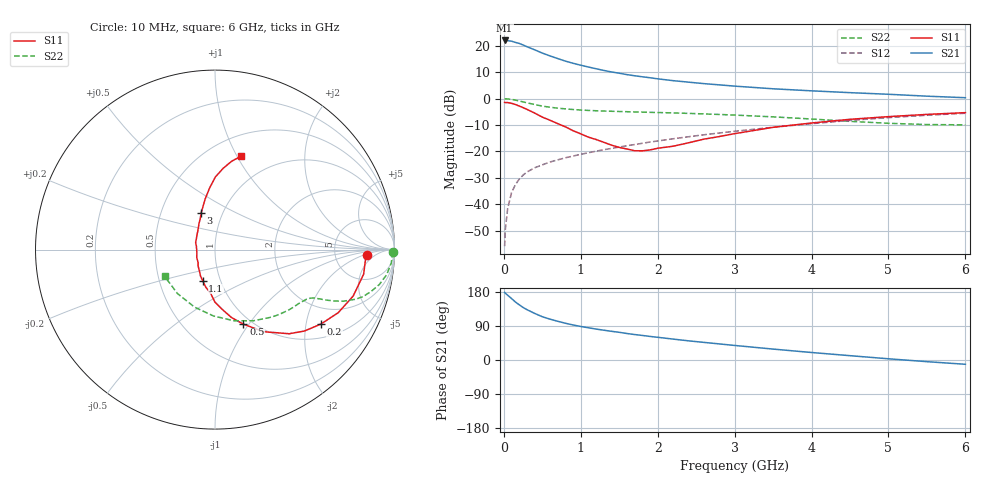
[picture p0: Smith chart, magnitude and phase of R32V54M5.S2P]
! SIEMENS Small Signal Semiconductors
! BFR181
! Si NPN RF Bipolar Junction Transistor in SOT23
! VCE = 2.5 V  IC = 4.5 mA
! Common Emitter S-Parameters:  May  1996
# GHz  S  MA  R  50
!  f  S11  S21  S12  S22
! GHz  MAG  ANG  MAG  ANG  MAG  ANG  MAG  ANG
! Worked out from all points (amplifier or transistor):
!   36 points, 10 MHz to 6 GHz, reference 50 ohm
!   highest |S21| = 22.0 dB at 10 MHz (marker M1)
!   |S21| within 3 dB of that: start of sweep to 354.1 MHz
!   unconditionally stable (mu >= 1): 1.156 GHz to 3.025 GHz
!   at 250 MHz: K = 0.39, MSG = 24.6 dB, |S12| = -29.0 dB
!   at 1.4 GHz: K = 1.05, MAG = 13.2 dB, |S12| = -18.9 dB
!   at 6 GHz: K = 0.86, MSG = 2.9 dB, |S12| = -5.6 dB
!   S11 on the Smith chart (normalised r, x): 10 MHz: 12, -2; 200 MHz: 1.41, -2.45; 500 MHz: 0.91, -0.94; 1.1 GHz: 0.82, -0.29; 3 GHz: 0.79, +0.34; 6 GHz: 0.71, +1.04
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0.01  0.8457 -1.9  12.61 178.2  0.0016 92.1  0.9919 -0.8
0.02  0.8404 -3.7  12.32 176.1  0.0034 87.3  0.9884 -1.7
0.05  0.8393 -9.4  12.48 170.9  0.0083 81.4  0.9852 -4.3
0.1  0.8121 -18.6  12.23 162.2  0.0165 81.3  0.9668 -8.3
0.15  0.7714 -27.1  11.57 153.1  0.0234 75.3  0.9359 -12.0
0.2  0.722 -35.0  11.09 145.7  0.0298 72.5  0.9005 -15.0
0.25  0.6739 -42.3  10.35 138.7  0.0355 69.3  0.8656 -17.6
0.3  0.625 -48.6  9.609 132.9  0.0406 67.5  0.8317 -19.4
0.4  0.5321 -59.3  8.388 123.0  0.0488 63.8  0.7711 -21.9
0.5  0.4451 -69.1  7.269 114.2  0.0555 62.5  0.7205 -23.4
0.6  0.3889 -76.4  6.427 107.8  0.0628 62.2  0.6847 -24.3
0.8  0.2918 -90.2  5.124 97.0  0.0755 61.7  0.6381 -25.4
0.9  0.2459 -95.5  4.662 92.4  0.0816 62.1  0.62 -25.8
1.1  0.1858 -111.7  3.959 85.0  0.0942 62.9  0.5962 -27.0
1.3  0.1484 -125.6  3.41 78.6  0.1075 63.1  0.5802 -28.4
1.6  0.1109 -156.3  2.843 69.9  0.1279 63.3  0.5638 -31.1
2.2  0.1251 144.4  2.184 55.2  0.1731 62.2  0.5348 -38.3
3  0.2165 111.0  1.721 38.4  0.2398 57.8  0.4868 -50.9
3.5  0.2855 101.2  1.532 28.8  0.286 53.9  0.4504 -61.7
4.5  0.4046 89.7  1.294 11.4  0.3856 43.8  0.3699 -91.3
5.5  0.5012 79.3  1.11 -4.4  0.483 31.1  0.3219 -130.5
6  0.541 74.3  1.038 -11.3  0.5271 24.0  0.3178 -152.1
